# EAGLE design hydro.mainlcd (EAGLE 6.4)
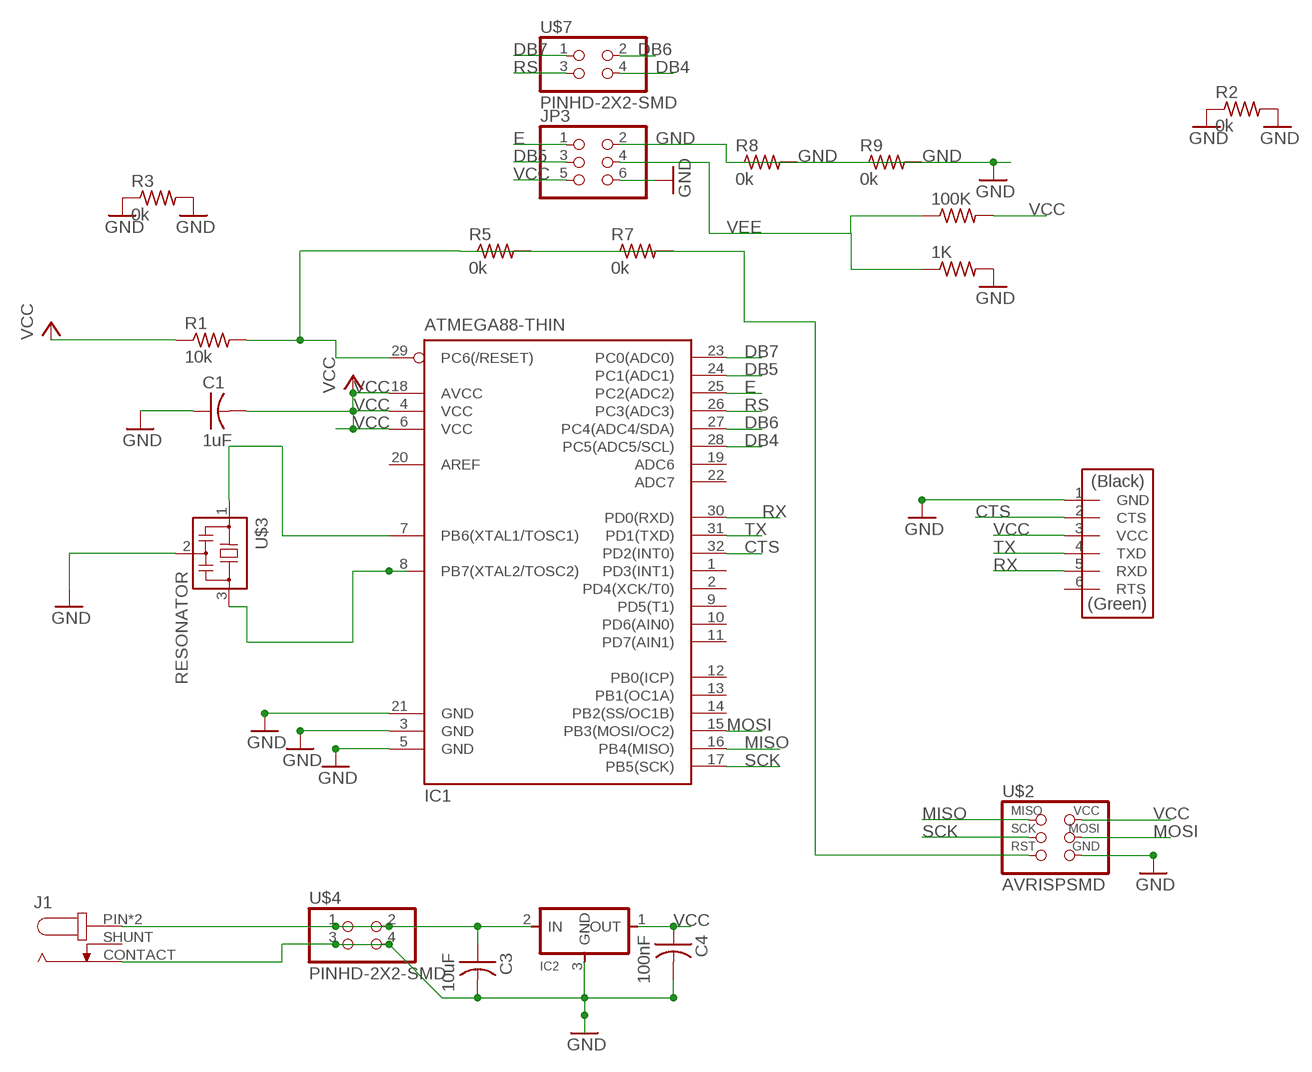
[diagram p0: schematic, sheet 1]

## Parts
1K  RES-US1206FAB  [R1206FAB]
100K  RES-US1206FAB  [R1206FAB]
C1  1uF  CAP-US1206FAB  [C1206FAB]
C3  10uF  CAP-US1206FAB  [C1206FAB]
C4  100nF  CAP-US1206FAB  [C1206FAB]
IC1  ATMEGA88-THIN  [TQFP32-08THIN]
IC2  REGULATORSOT23  [SOT23]
J1  JACK-PLUG  [JACK5.5]
JP3  PINHD-2X3-SMD  [2X03SMD]
R1  10k  RES-US1206FAB  [R1206FAB]
R2  0k  RES-US1206FAB  [R1206FAB]
R3  0k  RES-US1206FAB  [R1206FAB]
R5  0k  RES-US1206FAB  [R1206FAB]
R7  0k  RES-US1206FAB  [R1206FAB]
R8  0k  RES-US1206FAB  [R1206FAB]
R9  0k  RES-US1206FAB  [R1206FAB]
U$1  FTDI-SMD-HEADER  [1X06SMD]
U$2  AVRISPSMD  [2X03SMD]
U$3  RESONATOR  [EFOBM]
U$4  PINHD-2X2-SMD  [2X02SMD]
U$7  PINHD-2X2-SMD  [2X02SMD]

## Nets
CTS: IC1.32(PD2(INT0)) U$1.2(CTS)
DB4: IC1.28(PC5(ADC5/SCL)) U$7.4
DB5: IC1.24(PC1(ADC1)) JP3.3
DB6: IC1.27(PC4(ADC4/SDA)) U$7.2
DB7: IC1.23(PC0(ADC0)) U$7.1
E: IC1.25(PC2(ADC2)) JP3.1
GND: 1K.2 C1.1 C3.2 C4.2 IC1.3(GND) IC1.5(GND) IC1.21(GND) IC2.3(GND) J1.CONTACT JP3.2 JP3.6 R2.1 R2.2 R3.1 R3.2 R8.1 R8.2 R9.1 R9.2 U$1.1(GND) U$2.6(GND) U$3.2 U$4.3 U$4.4
MISO: IC1.16(PB4(MISO)) U$2.1(MISO)
MOSI: IC1.15(PB3(MOSI/OC2)) U$2.4(MOSI)
N$1: IC1.7(PB6(XTAL1/TOSC1)) U$3.1
N$2: IC1.8(PB7(XTAL2/TOSC2)) U$3.3
N$4: C3.1 IC2.2(IN) J1.PIN J1.PIN1(PIN) U$4.1 U$4.2
N$7: IC1.29(PC6(/RESET)) R1.2 R5.1 R5.2 R7.1 R7.2 U$2.5(RST)
RS: IC1.26(PC3(ADC3)) U$7.3
RX: IC1.30(PD0(RXD)) U$1.5(RXD)
SCK: IC1.17(PB5(SCK)) U$2.3(SCK)
TX: IC1.31(PD1(TXD)) U$1.4(TXD)
VCC: 100K.2 C1.2 C4.1 IC1.4(VCC) IC1.6(VCC) IC1.18(AVCC) IC2.1(OUT) JP3.5 R1.1 U$1.3(VCC) U$2.2(VCC)
VEE: 1K.1 100K.1 JP3.4
Unconnected: IC1.1(PD3(INT1)) IC1.2(PD4(XCK/T0)) IC1.9(PD5(T1)) IC1.10(PD6(AIN0)) IC1.11(PD7(AIN1)) IC1.12(PB0(ICP)) IC1.13(PB1(OC1A)) IC1.14(PB2(SS/OC1B)) IC1.19(ADC6) IC1.20(AREF) IC1.22(ADC7) J1.SHUNT U$1.6(RTS)

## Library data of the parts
1K 100K R1-R3 R5 R7-R9 = fab:RES-US: Resistor (US Symbol)
C1 C3 C4 = fab:CAP-US
IC1 = fab:ATMEGA88-THIN
IC2 = fab:REGULATOR
J1 = test:JACK-PLUG: DC POWER JACK Power Jack, DC, Right Angle, Through Hole, Rated 5A at 16VDC, PC Terminals Distributor: Farnell (www.Farnell.de) Drawing: 84N1161.pdf / 84N1162.pdf Manufacturer: SPC Technology (www.spctechnology.com) Type: SPC4077 / SPC 4078
JP3 = fab:PINHD-2X3-SMD: PIN HEADER
U$1 = fab:FTDI-SMD-HEADER
U$2 = fab:AVRISP
U$3 = fab:RESONATOR
U$4 U$7 = fab:PINHD-2X2-SMD

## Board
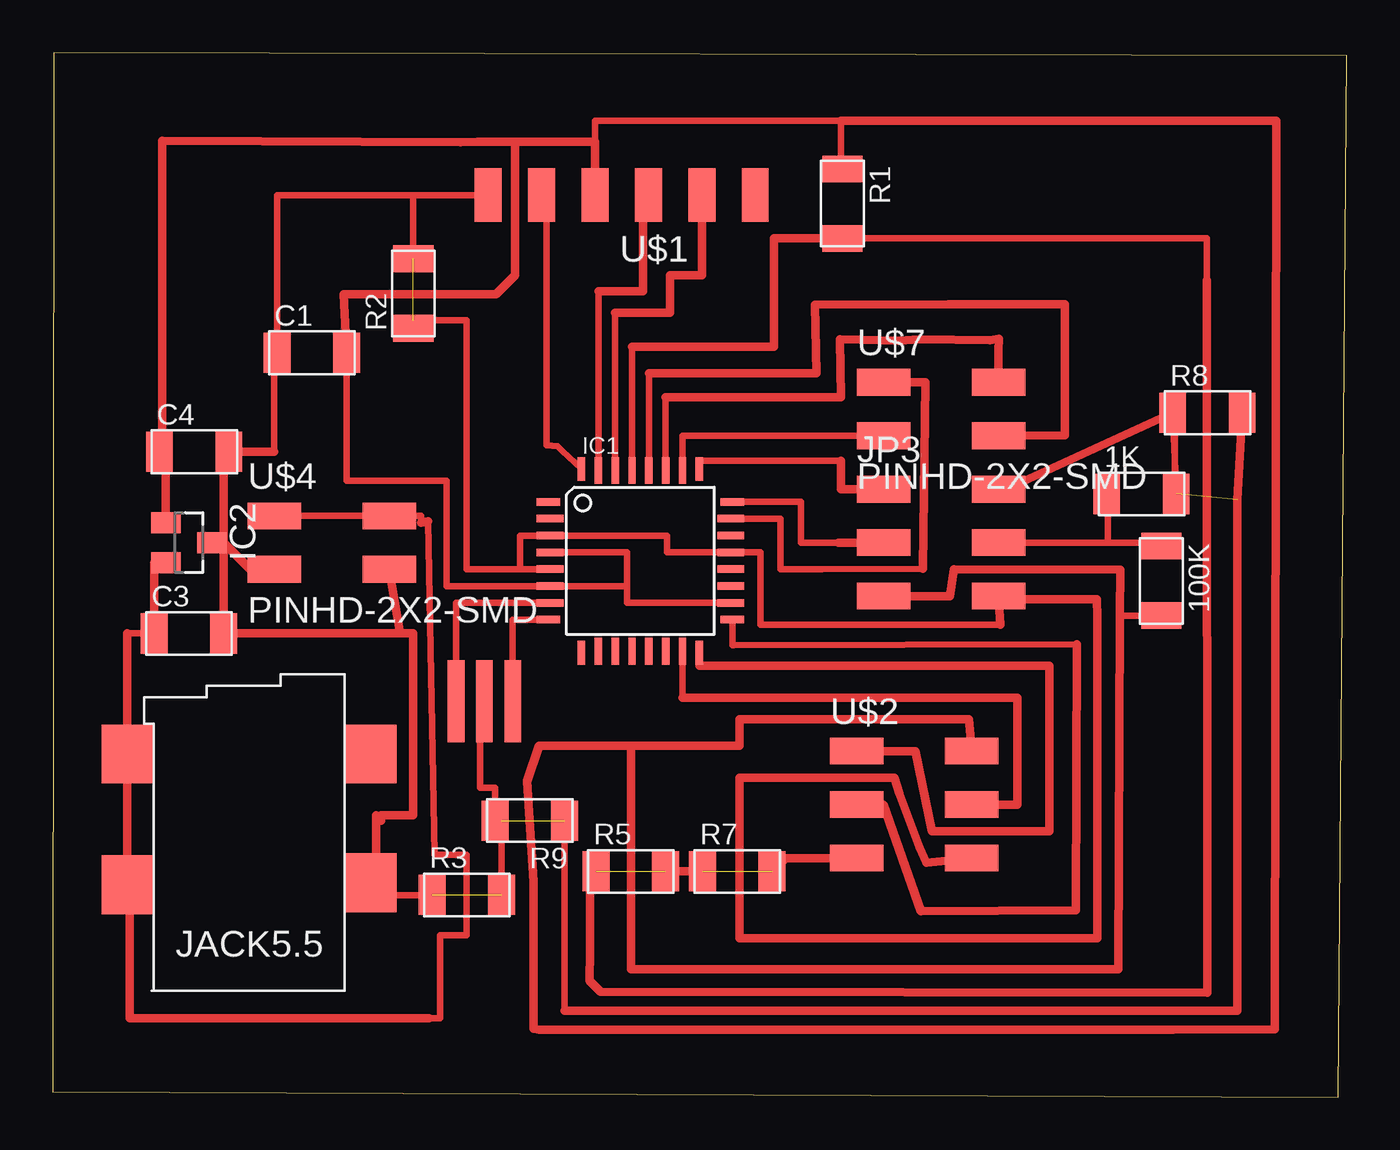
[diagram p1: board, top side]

Size 61.52 x 49.63 mm. Coordinates in mm from the lower left corner, seen from the top.
Outline: 0,0.27 61.1,0 61.52,49.48 0.05,49.63 0,0.27
Copper layers (1*16): Top 0.035mm / dielectric 1.5mm / Bottom 0.035mm
Design rules "default *": minimum track width 10mil, minimum drill 24mil, track to track 0.4mm, track to pad 0.41mm, pad to pad 0.41mm, via to via 0.41mm, smd to smd 8mil, copper to edge 40mil, drill to drill 8mil, minimum pad ring 10mil, minimum via ring 8mil, stop-mask expansion 4mil, vias tented up to drill 0mil, thermal gap 10mil

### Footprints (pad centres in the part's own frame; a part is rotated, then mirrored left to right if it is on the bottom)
R1206FAB = smd 1.27 x 1.905: 1 -1.651,0; 2 1.651,0
C1206FAB = smd 1.27 x 1.905: 1 -1.651,0; 2 1.651,0
TQFP32-08THIN = smd 1.118 x 0.356: 1 -4.369,2.8; 8 -4.369,-2.8; 17 4.369,-2.8; 24 4.369,2.8 | smd 1.27 x 0.356: 2 -4.293,2; 3 -4.293,1.2; 4 -4.293,0.4; 5 -4.293,-0.4; 6 -4.293,-1.2; 7 -4.293,-2; 18 4.293,-2; 19 4.293,-1.2; 20 4.293,-0.4; 21 4.293,0.4; 22 4.293,1.2; 23 4.293,2 | smd 0.356 x 1.118: 9 -2.8,-4.369; 16 2.8,-4.369; 25 2.8,4.369; 32 -2.8,4.369 | smd 0.356 x 1.27: 10 -2,-4.293; 14 1.2,-4.293; 15 2,-4.293; 26 2,4.293; 27 1.2,4.293; 31 -2,4.293 | smd 0.35 x 1.27: 11 -1.2,-4.293; 12 -0.4,-4.293; 13 0.4,-4.293; 28 0.4,4.293; 29 -0.4,4.293; 30 -1.2,4.293
SOT23 = smd 1 x 1.4: 1 -0.95,-1.1; 2 0.95,-1.1; 3 0,1.1
JACK5.5 = smd 2.4 x 2.8: CONTACT 10.58,6.06; PIN -1.03,12.18; PIN1 -1.03,5.97; SHUNT 10.58,12.18
2X03SMD = smd 2.54 x 1.27: 1 -2.54,2.54; 2 2.92,2.54; 3 -2.54,0; 4 2.92,0; 5 -2.54,-2.54; 6 2.92,-2.54
1X06SMD = smd 2.54 x 1.27: 1 0,6.35; 2 0,3.81; 3 0,1.27; 4 0,-1.27; 5 0,-3.81; 6 0,-6.35
EFOBM = smd 0.8 x 3.9: 1 -1.35,0; 2 0,0; 3 1.35,0
2X02SMD = smd 2.54 x 1.27: 1 -2.54,1.27; 2 2.92,1.27; 3 -2.54,-1.27; 4 2.92,-1.27

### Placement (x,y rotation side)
1K  51.75,28.66 0 top
100K  52.7,24.54 270 top
C1  12.32,35.37 0 top
C3  6.48,22.03 0 top
C4  6.73,30.67 0 top
IC1  27.94,25.49 0 top
IC2  6.48,26.35 270 top
J1  4.57,4.13 0 top
JP3  42.04,26.35 0 top
R1  37.54,42.46 270 top
R2  17.14,38.19 90 top
R3  19.68,9.61 0 top
R5  27.48,10.73 0 top
R7  32.54,10.73 0 top
R8  54.89,32.52 0 top
R9  22.68,13.14 180 top
U$1  27.05,42.86 90 top
U$2  40.77,13.91 0 top
U$3  20.52,18.81 0 top
U$4  13.08,26.35 0 top
U$7  42.04,32.7 0 top

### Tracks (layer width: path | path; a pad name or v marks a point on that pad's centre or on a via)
CTS
  Top 0.305: IC1.32 24.21,30.72 24,30.92 23.48,30.97 23.48,41.85 23.5,41.85
  Top 0.406: U$1.2 23.5,41.85
DB4
  Top 0.305: IC1.28 28.34,34.4
  Top 0.406: U$7.4 48.11,31.46 48.11,37.68 42.57,37.68 36.25,37.66 36.3,34.4 28.57,34.4 28.47,34.4 28.34,34.4
DB5
  Top 0.305: IC1.24 35.56,28.29 35.56,26.35 37.36,26.35
  Top 0.406: 37.36,26.35 JP3.3
DB6
  Top 0.305: IC1.27 29.14,33.26
  Top 0.406: 45.62,33.85 U$7.2 44.96,35.47 44.98,36.03 44.55,35.98 41.2,36 40.23,35.95 37.41,36 37.47,33.26 29.14,33.26
DB7
  Top 0.305: 41.38,25.11 36.58,25.08 34.61,25.08 34.61,27.49 IC1.23
  Top 0.406: U$7.1 41.48,33.97 41.38,25.11
E
  Top 0.305: 37.47,30.24 30.74,30.24 IC1.25
  Top 0.406: 37.47,30.24 37.47,28.89 JP3.1
GND  (4 unrouted)
  Top 0.305: 45.06,22.44 33.66,22.44 33.66,25.89 IC1.21 29.21,25.89 29.21,26.69 IC1.3 22.23,26.69 22.23,25.09 | IC1.5 22.23,25.09 | 10.54,30.67 10.54,34.73 C1.1 10.67,42.86 17.14,42.86 | U$1.1 17.14,42.86 | 22.23,25.09 19.68,25.09 19.68,36.92 17.14,36.92 R2.1 | R2.2 17.14,42.86 | U$3.2 20.32,18.81 20.32,14.69 21.03,14.69 R9.2 21.34,13.14 R3.2 | 9.4,25.08 U$4.3 | R3.1 18.03,9.59 15.37,9.59 15.15,9.59 J1.CONTACT | 24.33,4.1 R9.1 | R8.1 53.24,32.47 1K.2 53.34,28.66 53.34,31.84
  Top 0.406: U$2.6 41.53,11.14 41.2,11.87 40.26,14.41 40.01,15.18 32.64,15.18 32.64,7.56 49.66,7.56 49.66,22.8 49.63,23.66 45.21,23.66 45.21,23.74 44.96,23.74 JP3.6 45.06,22.44 | IC2.3 8.13,26.35 | 8.13,26.35 C3.2 16.51,22.03 | 15.37,13.4 15.37,13.14 | 8.13,26.35 8.13,30.67 C4.2 10.54,30.67 | 15.37,13.14 15.62,13.14 15.62,13.4 17.14,13.4 17.14,22.03 16.51,22.03 | 15.37,13.14 15.37,9.59 | 16.51,22.03 U$4.4 | 8.13,26.35 9.4,25.08 | JP3.2 44.96,28.71 R8.1 | R8.2 56.31,28.4 56.31,4.1 24.33,4.1
MISO
  Top 0.305: IC1.16 30.74,20.49
  Top 0.406: U$2.1 41.02,16.45 41.78,12.64 47.37,12.64 47.37,20.51 31.45,20.49 30.74,20.49
MOSI
  Top 0.305: IC1.15 29.94,18.99
  Top 0.406: U$2.4 45.85,13.91 45.85,18.99 29.94,18.99
N$1
  Top 0.305: U$3.1 19.17,23.49 IC1.7
N$2
  Top 0.305: U$3.3 21.87,22.69 IC1.8
N$4
  Top 0.305: 17.91,3.75 18.41,3.75 18.41,7.71 19.68,7.71 19.68,11.52 18.16,11.52 17.84,27.37 | U$4.1 U$4.2 17.53,27.62 17.53,27.3 | 3.54,22.03 C3.1
  Top 0.406: 17.53,27.3 17.84,27.37 | 17.91,3.75 3.68,3.75 3.67,3.76 3.67,10.1 J1.PIN1 J1.PIN 3.54,22.03 | C3.1 4.83,25.4 IC2.2 5.46,25.4 5.46,25.34
N$7  (2 unrouted)
  Top 0.305: IC1.29 27.54,35.65 | R1.2 54.87,40.8 54.87,38.82
  Top 0.406: 27.54,35.65 34.29,35.65 34.29,40.8 R1.2 | 54.87,38.82 54.89,4.97 26.04,5.02 25.53,5.52 25.55,6.97 25.55,10.83 R5.1 | R5.2 R7.1 | R7.2 34.82,11.37 U$2.5
RS
  Top 0.305: IC1.26 29.94,31.43 U$7.3
RX
  Top 0.305: IC1.30 26.74,37.27
  Top 0.406: U$1.5 30.86,39.05 29.34,39.05 29.34,37.27 27.3,37.27 26.87,37.27 26.74,37.27
SCK
  Top 0.305: 48.69,21.53 32.36,21.48 32.31,21.48 IC1.17
  Top 0.406: U$2.3 39.5,13.91 41.27,8.83 48.64,8.88 48.69,21.53
TX
  Top 0.305: IC1.31 25.94,38.29
  Top 0.406: U$1.4 28.07,42.1 28.07,38.29 25.94,38.29
VCC
  Top 0.305: IC1.18 27.3,23.49 27.3,24.29 | 27.3,24.29 IC1.6 18.73,24.29 18.73,29.3 13.97,29.3 C1.2 | 27.3,24.29 27.3,25.89 IC1.4 | R1.1 37.47,44.11 37.47,46.41 25.78,46.41 25.78,45.4 | 100K.2 50.74,22.89 50.74,22.95
  Top 0.406: U$1.3 25.78,45.4 21.97,45.4 | 21.97,45.4 20.19,45.4 19.38,45.38 5.21,45.45 5.21,30.67 | C4.1 5.21,30.67 | IC2.1 5.38,30.67 5.21,30.67 | U$2.2 43.56,17.97 32.64,17.97 32.64,16.7 27.48,16.7 | 27.48,16.7 23.11,16.7 22.54,15.01 22.86,10.25 22.86,3.26 23.11,3.21 53.26,3.21 58.09,3.24 58.17,46.39 37.47,46.41 | C1.2 13.84,38.16 21.08,38.16 21.97,39.05 21.97,45.4 | JP3.5 42.65,23.81 42.85,25.08 50.75,25.06 50.74,22.95 50.65,6.08 27.48,6.08 27.48,16.7
VEE
  Top 0.305: JP3.4 50.16,26.35 | 50.16,26.35 52.7,26.35 100K.1 | 1K.1 50.16,28.66 50.16,26.35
